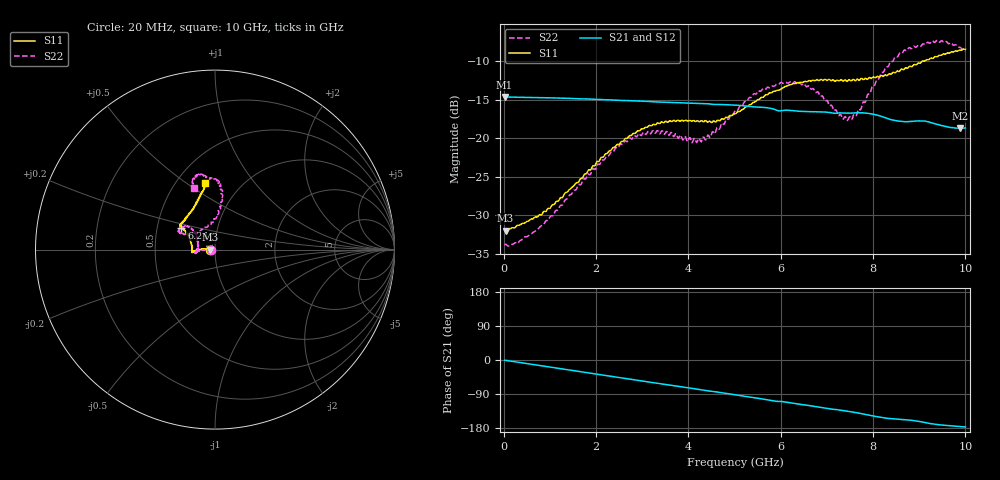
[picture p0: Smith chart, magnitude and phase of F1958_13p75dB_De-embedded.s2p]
! Integrated Device Technology
! Corporate Headquarters
! 6024 Silver Creek Valley Road
! San Jose, CA 95138  USA
! Phone:  1-408-284-8200
! Toll Free:  1-800-223-1366
! Webpage:  http://www.idt.com/
! Timing and RF Division
! 515 Groton Road, Suite 102
! Westford, MA 01886-6024
! Device:  F1958
! Description: 7-bit 0.25 dB Digital Step Attenuator
! Frequency:  0.001 -  6.000 GHz
! Package:  4x4 mm Thin QFN Plastic Package: 24 pin
! Ports:  2 RF, 12 DC
!  Pin  1  = D0
!  Pin  2  = VDD
!  Pin  3  = VMODE
!  Pin  4  = GND
!  Pin  5  = RF1  =  Port 1
!  Pin  6  = GND
!  Pin  7  = GND
!  Pin  8  = GND
!  Pin  9  = GND
!  Pin 10  = GND
!  Pin 11  = GND
!  Pin 12  = GND
!  Pin 13  = GND
!  Pin 14  = RF2  =  Port 2
!  Pin 15  = GND
!  Pin 16  = LE
!  Pin 17  = CLK
!  Pin 18  = DATA
!  Pin 19  = D6
!  Pin 20  = D5
!  Pin 21  = D4
!  Pin 22  = D3
!  Pin 23  = D2
!  Pin 24  = D1
! State:  55
! Atten State:  13.75 dB
! Voltage:  +3.30 Volts
! Current:  0.258 mA
! Data:  The device was measured on a F1958 evaluation board which has
!  individual transmission lines to the RF pins.  Data was collected
!  using a calibrated network analyzer.  The evaluation board was
!  de-embedded using Automatic Fixture Removal (AFR).
!  The reference plane is the edge of the package pin.
! Misc:
!  Action Tracker AT0419
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# GHz S dB R 50
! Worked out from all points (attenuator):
!   500 points, 20 MHz to 10 GHz, reference 50 ohm
!   highest |S21| = -14.65 dB at 20 MHz (marker M1); lowest = -18.7 dB at 9.88 GHz (marker M2)
!   lowest |S11| = -32.0 dB at 40 MHz (marker M3), VSWR 1.05, Z = 47.6 - j0.0761 ohm
!   |S11| at or under -10 dB: start of sweep to 9.073 GHz; 9.090293 GHz to 9.120818 GHz (30.53 MHz wide, 0.335 % of centre)
!   |S22| runs from -34.0 to -7.3 dB; largest |S21 - S12| = 0.00057
!   S11 on the Smith chart (normalised r, x): 20 MHz: 0.95, -0.00; 6.24 GHz: 0.67, +0.17; 10 GHz: 0.69, +0.60
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0.02  -31.98 -178.1  -14.65 -0.5  -14.65 -0.5  -33.87 -177.8
0.04  -32.00 -178.2  -14.66 -0.9  -14.66 -0.9  -33.79 -176.8
0.32  -31.32 177.5  -14.71 -6.2  -14.70 -6.1  -33.56 179.3
0.72  -30.26 177.2  -14.75 -13.6  -14.74 -13.6  -31.90 -179.5
1.7  -25.21 177.4  -14.91 -31.7  -14.91 -31.6  -25.65 -179.7
2.6  -20.33 -178.8  -15.12 -48.1  -15.10 -48.1  -20.60 -175.7
2.92  -19.06 -176.0  -15.19 -54.0  -15.18 -54.1  -19.44 -172.6
3.36  -18.11 -173.6  -15.32 -62.0  -15.32 -62.1  -19.30 -168.7
4.24  -17.89 -178.7  -15.50 -77.7  -15.52 -77.8  -20.08 169.0
4.5  -17.98 175.5  -15.61 -82.7  -15.62 -82.7  -19.52 153.5
5.02  -16.85 160.8  -15.72 -91.9  -15.73 -91.9  -16.36 139.6
5.54  -14.96 150.6  -15.98 -101.6  -16.00 -101.6  -13.90 140.6
6.24  -13.02 146.7  -16.42 -113.8  -16.45 -113.8  -12.87 151.7
6.68  -12.52 144.9  -16.58 -121.3  -16.60 -121.2  -13.63 153.5
7.3  -12.42 138.9  -16.74 -132.5  -16.74 -132.4  -16.91 132.3
7.5  -12.47 136.3  -16.76 -136.2  -16.76 -136.1  -17.26 114.2
7.68  -12.42 133.3  -16.71 -139.9  -16.71 -139.8  -16.30 97.5
8.34  -11.69 117.6  -17.51 -154.2  -17.51 -154.4  -10.59 82.0
8.68  -11.01 110.8  -17.87 -157.5  -17.87 -157.5  -8.55 86.3
9.26  -9.61 102.9  -18.01 -168.0  -18.01 -168.2  -7.50 99.1
9.88  -8.57 98.6  -18.73 -175.5  -18.77 -175.4  -8.21 108.3
10  -8.49 98.3  -18.68 -176.8  -18.72 -176.7  -8.76 108.9
